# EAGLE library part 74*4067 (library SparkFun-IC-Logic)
16-channel analog MUX Datasheet SparkFun Products MP3 Trigger (WIG-13720) SparkFun Analog/Digital MUX Breakout - CD74HC4067 (BOB-09056)
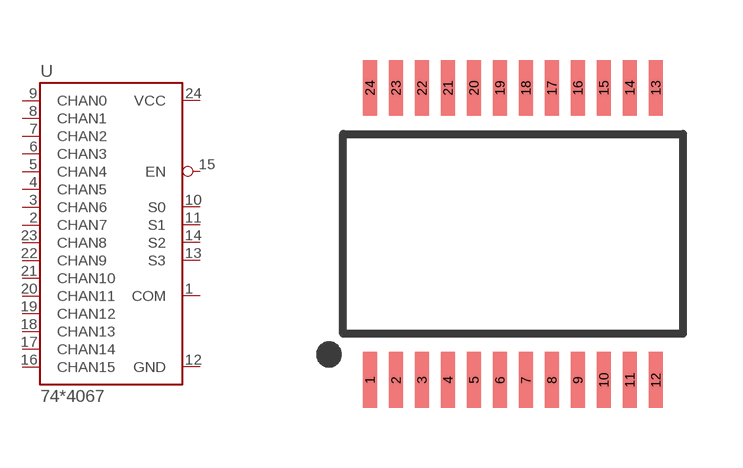
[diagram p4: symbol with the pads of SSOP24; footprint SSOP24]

Designator prefix U

## 74HC4067SM96 (PROD_ID: IC-08252; VALUE: CD74HC4067SM96)  [SSOP24]
1  COM
2  CHAN7
3  CHAN6
4  CHAN5
5  CHAN4
6  CHAN3
7  CHAN2
8  CHAN1
9  CHAN0
10  S0  in
11  S1  in
12  GND
13  S3  in
14  S2  in
15  EN  in
16  CHAN15
17  CHAN14
18  CHAN13
19  CHAN12
20  CHAN11
21  CHAN10
22  CHAN9
23  CHAN8
24  VCC

## Footprint SSOP24 (pad centres in mm)
smd 0.348 x 1.397: 1 -3.575,-3.656; 2 -2.925,-3.656; 3 -2.275,-3.656; 4 -1.625,-3.656; 5 -0.975,-3.656; 6 -0.325,-3.656; 7 0.325,-3.656; 8 0.975,-3.656; 9 1.625,-3.656; 10 2.275,-3.656; 11 2.925,-3.656; 12 3.575,-3.656; 13 3.575,3.656; 14 2.925,3.656; 15 2.275,3.656; 16 1.625,3.656; 17 0.975,3.656; 18 0.325,3.656; 19 -0.325,3.656; 20 -0.975,3.656; 21 -1.625,3.656; 22 -2.275,3.656; 23 -2.925,3.656; 24 -3.575,3.656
